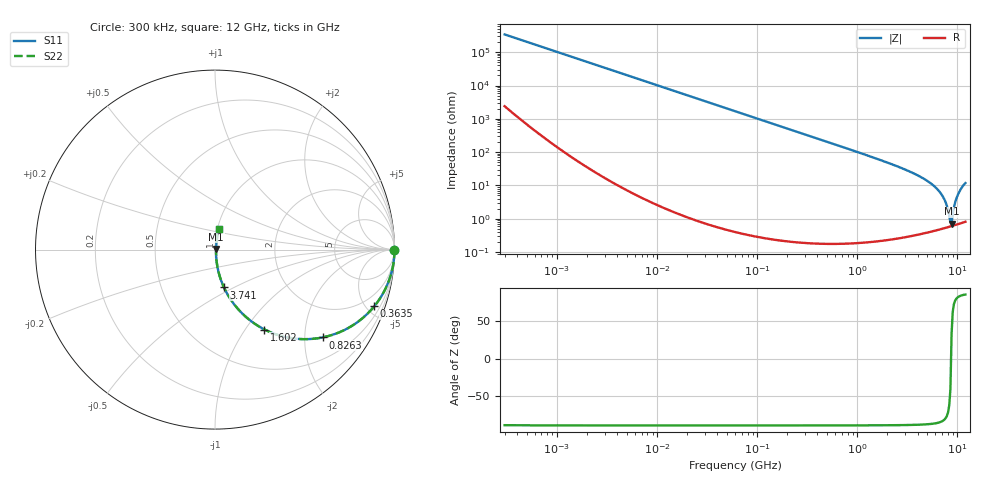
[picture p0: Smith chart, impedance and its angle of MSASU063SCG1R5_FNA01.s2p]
! MSASU063SCG1R5_FNA01  S-PARAMETER MODEL  ( Standard Model )
! Model Generated by TAIYO YUDEN Corporation (http://www.ty-top.com)
! Version 1.0
! TAIYO YUDEN Control No. 240819
! Copyright(c) 2024 TAIYO YUDEN CO.,LTD. All Rights Reserved.
! Product Description (link to TY-COMPAS)
! https://ds.yuden.co.jp/TYCOMPAS/or/detail?pn=MSASU063SCG1R5CFNA01&u=M
! Products Name : Multilayer Ceramic Capacitors
! Characteristics :
!  Capacitance : 1.5 [pF] , Rated Voltage : 50 [V] , TCC : CG / C0G
!  Case Size : 0.6 x 0.3 / 0.024 x 0.012 [mm/inch] , Thickness : 0.3 / 0.012 [mm/inch]
!  (Conditions: Temperature = 25 [degC] , DC Bias Voltage = 0 [V])
! External Node Assignments :
!  1  o---| |---o  2
! GND o---------o GND
! Frequency Range : 0.3MHz  -  12000MHz  [ 401 STEP ]
# MHZ S RI R 50
! Freq[MHz].  S11 Real  S11 Imag  S21 Real  S21 Imag  S12 Real  S12 Imag  S22 Real  S22 Imag
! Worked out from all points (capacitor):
!   401 points, 300 kHz to 12 GHz, reference 50 ohm
!   read as one part in series: C = 1.56 pF near 316.3 kHz
!   lowest |Z| = 712 mohm at 8.732 GHz (marker M1)
!   series resonance near 8.634 GHz, so ESL is about 220 pH
!   S11 on the Smith chart (normalised r, x): 300 kHz: open; 363.5 MHz: 1.00, -5.61; 826.3 MHz: 1.00, -2.45; 1.602 GHz: 1.00, -1.23; 3.741 GHz: 1.01, -0.44; 12 GHz: 1.02, +0.24
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0.3  1 -0.000294  2.14e-06 0.000294  2.14e-06 0.000294  1 -0.000294
1.769972  1 -0.00173  4.33e-06 0.00173  4.33e-06 0.00173  1 -0.00173
10.44266  0.9999 -0.0102  0.000107 0.0102  0.000107 0.0102  0.9999 -0.0102
60  0.9966 -0.0585  0.00345 0.0585  0.00345 0.0585  0.9966 -0.0585
155.7172  0.9772 -0.149  0.0228 0.149  0.0228 0.149  0.9772 -0.149
353.9943  0.8924 -0.3096  0.1076 0.3096  0.1076 0.3096  0.8924 -0.3096
363.4975  0.8872 -0.3161  0.1128 0.3161  0.1128 0.3161  0.8872 -0.3161
826.3444  0.6001 -0.4891  0.3999 0.4891  0.3999 0.4891  0.6001 -0.4891
1602.47  0.2757 -0.4452  0.7243 0.4452  0.7243 0.4452  0.2757 -0.4452
2088.533  0.1765 -0.3787  0.8235 0.3787  0.8235 0.3787  0.1765 -0.3787
3740.715  0.0499 -0.2107  0.9501 0.2107  0.9501 0.2107  0.0499 -0.2107
5140.631  0.0201 -0.126  0.9799 0.126  0.9799 0.126  0.0201 -0.126
6524.734  0.00922 -0.0672  0.9908 0.0672  0.9908 0.0672  0.00922 -0.0672
7448.838  0.00648 -0.0357  0.9935 0.0357  0.9935 0.0357  0.00648 -0.0357
7854.144  0.00598 -0.0233  0.994 0.0233  0.994 0.0233  0.00598 -0.0233
8281.503  0.00581 -0.0109  0.9942 0.0109  0.9942 0.0109  0.00581 -0.0109
8732.115  0.00597 0.0038  0.994 -0.0038  0.994 -0.0038  0.00597 0.0038
8966.534  0.00624 0.0117  0.9938 -0.0117  0.9938 -0.0117  0.00624 0.0117
9708.23  0.00799 0.0377  0.992 -0.0377  0.992 -0.0377  0.00799 0.0377
10236.47  0.0101 0.0561  0.9899 -0.0561  0.9899 -0.0561  0.0101 0.0561
11083.22  0.0148 0.0853  0.9852 -0.0853  0.9852 -0.0853  0.0148 0.0853
12000  0.0214 0.1143  0.9786 -0.1143  0.9786 -0.1143  0.0214 0.1143
